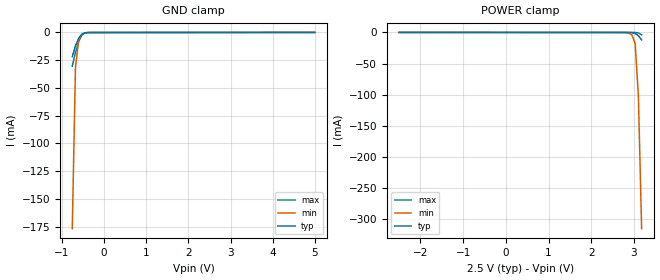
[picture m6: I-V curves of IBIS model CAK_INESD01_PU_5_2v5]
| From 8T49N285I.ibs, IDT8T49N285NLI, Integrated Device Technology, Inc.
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[Model] CAK_INESD01_PU_5_2v5
Model_type   Input
Polarity   Non-Inverting
Vinl = 0.7V
Vinh = 1.7V
|   typ   min   max
C_comp   2pF   1.5pF   2.5pF
|   typ   min   max
[Voltage range]   2.5V   2.375V   2.625V
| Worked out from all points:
|   GND clamp passes 1 mA (typ) near -0.50 V on its own axis
[GND_clamp]
|Voltage   I (typ)   I (min)   I (max)
|Note, modeling breaks down at 250mA and above.  This is well beyond the functional   |
|operating range of the device.  Should this scenario occur, catastrophic failure and   |
|possible damage to the device and/or board is of higher concern than the I-V curve   |
|behavior.  The IBIS checker will flag currents in excess of 10A with warnings.  Lines   |
|with currents in excess of 0.35 A have been commented out.  The points still remain|
|available to the user if the user desires to use them.   |
|-2.50000e+00   -6.31282e+00   -5.12663e+00   -7.65740e+00
|-2.42424e+00   -6.02358e+00   -4.91001e+00   -7.28826e+00
|-2.34848e+00   -5.73437e+00   -4.69348e+00   -6.91913e+00
|-2.27273e+00   -5.44522e+00   -4.47703e+00   -6.55002e+00
|-2.19697e+00   -5.15613e+00   -4.26068e+00   -6.18093e+00
|-2.12121e+00   -4.86711e+00   -4.04442e+00   -5.81188e+00
|-2.04545e+00   -4.57816e+00   -3.82827e+00   -5.44287e+00
|-1.96970e+00   -4.28929e+00   -3.61222e+00   -5.07391e+00
|-1.89394e+00   -4.00052e+00   -3.39629e+00   -4.70501e+00
|-1.81818e+00   -3.71186e+00   -3.18049e+00   -4.33619e+00
|-1.74242e+00   -3.42332e+00   -2.96481e+00   -3.96746e+00
|-1.66667e+00   -3.13491e+00   -2.74927e+00   -3.59882e+00
|-1.59091e+00   -2.84666e+00   -2.53388e+00   -3.23029e+00
|-1.51515e+00   -2.55857e+00   -2.31863e+00   -2.86189e+00
|-1.43939e+00   -2.27067e+00   -2.10354e+00   -2.49363e+00
|-1.36364e+00   -1.98298e+00   -1.88861e+00   -2.12553e+00
|-1.28788e+00   -1.69551e+00   -1.67386e+00   -1.75764e+00
|-1.21212e+00   -1.40830e+00   -1.45928e+00   -1.38998e+00
|-1.13636e+00   -1.12135e+00   -1.24489e+00   -1.02259e+00
|-1.06061e+00   -8.34691e-01   -1.03071e+00   -6.55507e-01
|-9.84848e-01   -5.48353e-01   -8.16770e-01   -2.88773e-01
|-9.09091e-01   -2.62364e-01   -6.03157e-01   -6.18867e-02
|-8.33333e-01   -5.03221e-02   -3.90013e-01   -4.20161e-02
-757.6mV  -21.82mA   -176.9mA   -30.35mA
-681.8mV  -11.99mA   -31.47mA   -18.03mA
-606.1mV  -5.287mA   -6.69mA    -8.181mA
-530.3mV  -1.547mA   -1.657mA   -2.318mA
-454.5mV  -303.7uA   -377.6uA   -387.1uA
-378.8mV  -83.09uA   -102uA     -93.25uA
5V        49.8uA     45.82uA    54.66uA
[Power_clamp]
|Voltage   I (typ)   I (min)   I (max)
|Note, modeling breaks down at 250mA and above.  This is well beyond the functional   |
|operating range of the device.  Should this scenario occur, catastrophic failure and   |
|possible damage to the device and/or board is of higher concern than the I-V curve   |
|behavior.  The IBIS checker will flag currents in excess of 10A with warnings.  Lines   |
|with currents in excess of 0.35 A have been commented out.  The points still remain|
|available to the user if the user desires to use them.   |
-2.5V     49.8uA     43.64uA    57.54uA
2.727V    -54.43uA   -75.06uA   -62.76uA
2.879V    -83.09uA   -997.4uA   -66.35uA
2.955V    -303.7uA   -4.106mA   -71.16uA
3.03V     -1.547mA   -17.66mA   -133.7uA
3.106V    -5.287mA   -102.4mA   -746.9uA
3.182V    -11.99mA   -315.5mA   -3.861mA
